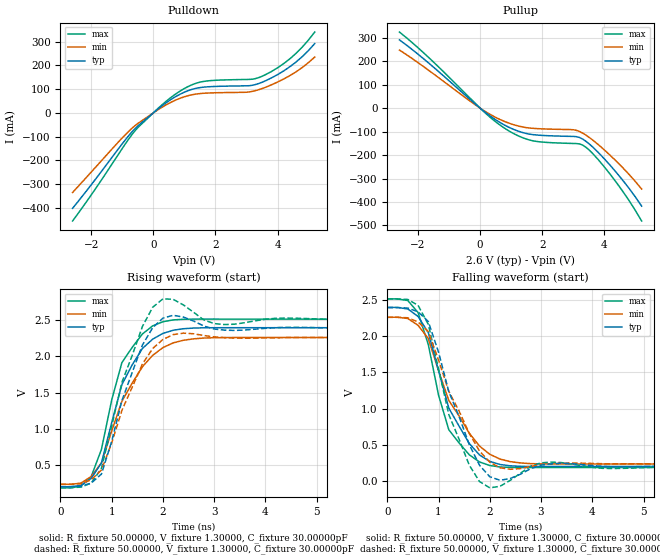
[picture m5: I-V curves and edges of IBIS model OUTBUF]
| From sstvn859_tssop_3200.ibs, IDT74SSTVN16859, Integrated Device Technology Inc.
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|   Model OUTBUF
[Model]   OUTBUF
Model_type   Output
Polarity   Inverting
Vmeas =  1.30000V
Cref = 30.00000pF
Rref =  50.00000
Vref =  1.30000V
C_comp   3.50000pF   3.50000pF   3.50000pF
[Temperature Range]   25.00000   70.00000   0.000
[Voltage Range]   2.60000V   2.50000V   2.70000V
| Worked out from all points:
|   slope of the pulldown table from 0 to 0.39 V, typ, clamps not added: 9.64 ohm
|   slope of the pullup table from 0 to 0.39 V, typ, clamps not added: 9.79 ohm
|   rising waveform, R_fixture 50.00000, V_fixture 1.30000, C_fixture 30.00000pF: 20-80 % time 626ps typ, 749ps min, 562ps max; typ from 0.202 V to 2.4 V
|   rising waveform, R_fixture 50.00000, V_fixture 1.30000, C_fixture 30.00000pF: 20-80 % time 576ps typ, 663ps min, 550ps max; typ from 0.204 V to 2.39 V
|   falling waveform, R_fixture 50.00000, V_fixture 1.30000, C_fixture 30.00000pF: 20-80 % time 663ps typ, 772ps min, 535ps max; typ from 2.4 V to 0.202 V
|   falling waveform, R_fixture 50.00000, V_fixture 1.30000, C_fixture 30.00000pF: 20-80 % time 612ps typ, 707ps min, 518ps max; typ from 2.39 V to 0.204 V
[Pulldown]
| voltage   I(typ)   I(min)   I(max)
-2.6V     -401.8mA   -335.1mA   -455.1mA
-1.8V     -268.7mA   -220.3mA   -307.6mA
-1V       -130mA     -105.2mA   -149.9mA
-600mV    -67.49mA   -54.84mA   -76.8mA
500mV     50.5mA     40.02mA    58.04mA
1V        87.18mA    67.84mA    102.6mA
1.5V      106.4mA    81.32mA    129.3mA
3.1V      114.6mA    88.34mA    141mA
3.6V      134.4mA    107.1mA    160mA
4.4V      194.5mA    157.1mA    227.9mA
4.8V      237.2mA    191.4mA    277.4mA
5.2V      291.9mA    235.2mA    340.4mA
[Pullup]
| voltage   I(typ)   I(min)   I(max)
-2.6V     291.1mA    247.9mA    324.7mA
-1.6V     185.9mA    155.8mA    208.8mA
0V        -2.777nA   -2.095nA   -2.207nA
900mV     -79.93mA   -62.64mA   -94.98mA
1.7V      -112.9mA   -85.98mA   -139.3mA
3V        -120.6mA   -92.11mA   -150.6mA
3.2V      -125.1mA   -99.61mA   -152.5mA
3.4V      -140.7mA   -114.5mA   -166.2mA
3.8V      -188.5mA   -155mA     -219.1mA
4.2V      -245.7mA   -202.7mA   -284.2mA
4.8V      -342.9mA   -283.3mA   -395.1mA
5.2V      -417.8mA   -345mA     -481.3mA
[Ramp]
| variable   typ   min   max
dV/dt_r   1.30200/0.16320n   1.19520/0.19481n   1.38720/0.12588n
dV/dt_f   1.30626/0.15532n   1.20012/0.19309n   1.38660/0.14172n
R_load = 50.00000
[Rising Waveform]
R_fixture = 50.00000
V_fixture = 1.30000
V_fixture_min = 1.25000
V_fixture_max = 1.35000
C_fixture = 30.00000pF
| time   V(typ)   V(min)   V(max)
0s        202.5mV    235.9mV    188mV
400ps     221.7mV    253.5mV    213.5mV
600ps     316.9mV    344.3mV    342.8mV
800ps     531.1mV    531.3mV    717.9mV
1ns       1.087V     971.4mV    1.398V
1.2ns     1.612V     1.382V     1.915V
1.6ns     2.109V     1.857V     2.309V
2ns       2.317V     2.121V     2.478V
3ns       2.395V     2.257V     2.514V
10ns      2.395V     2.26V      2.513V
[Rising Waveform]
R_fixture = 50.00000
V_fixture = 1.30000
V_fixture_min = 1.25000
V_fixture_max = 1.35000
C_fixture = 30.00000pF
R_dut = 0.10500
L_dut = 3.80000nH
C_dut = 0.22000pF
| time   V(typ)   V(min)   V(max)
0s        204.4mV    237.6mV    190.1mV
600ps     253.3mV    298.4mV    253.3mV
800ps     378mV      433.1mV    456.7mV
1.2ns     1.392V     1.256V     1.644V
1.6ns     2.156V     1.895V     2.412V
2ns       2.526V     2.233V     2.792V
2.4ns     2.542V     2.32V      2.708V
3.2ns     2.362V     2.259V     2.438V
4.4ns     2.4V       2.259V     2.528V
10ns      2.393V     2.258V     2.511V
[Falling Waveform]
R_fixture = 50.00000
V_fixture = 1.30000
V_fixture_min = 1.25000
V_fixture_max = 1.35000
C_fixture = 30.00000pF
| time   V(typ)   V(min)   V(max)
0s        2.395V     2.26V      2.513V
400ps     2.373V     2.242V     2.49V
600ps     2.271V     2.149V     2.324V
800ps     2.047V     1.965V     1.882V
1ns       1.522V     1.521V     1.184V
1.2ns     1.006V     1.112V     707.7mV
1.6ns     517.7mV    660mV      362.2mV
2ns       271.6mV    369.3mV    214.7mV
2.8ns     201.6mV    240.6mV    187mV
10ns      202.5mV    235.9mV    188mV
[Falling Waveform]
R_fixture = 50.00000
V_fixture = 1.30000
V_fixture_min = 1.25000
V_fixture_max = 1.35000
C_fixture = 30.00000pF
R_dut = 0.10500
L_dut = 3.80000nH
C_dut = 0.22000pF
| time   V(typ)   V(min)   V(max)
0s        2.393V     2.258V     2.511V
600ps     2.335V     2.195V     2.424V
800ps     2.2V       2.06V      2.161V
1.2ns     1.233V     1.236V     917.3mV
1.6ns     501.8mV    656.2mV    219.5mV
2ns       59.73mV    260.4mV    -93.3mV
2.4ns     35.61mV    162.5mV    10.94mV
3.2ns     237.7mV    236.6mV    261.7mV
4.4ns     196.3mV    237.1mV    173.2mV
10ns      204.4mV    237.6mV    190.1mV
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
